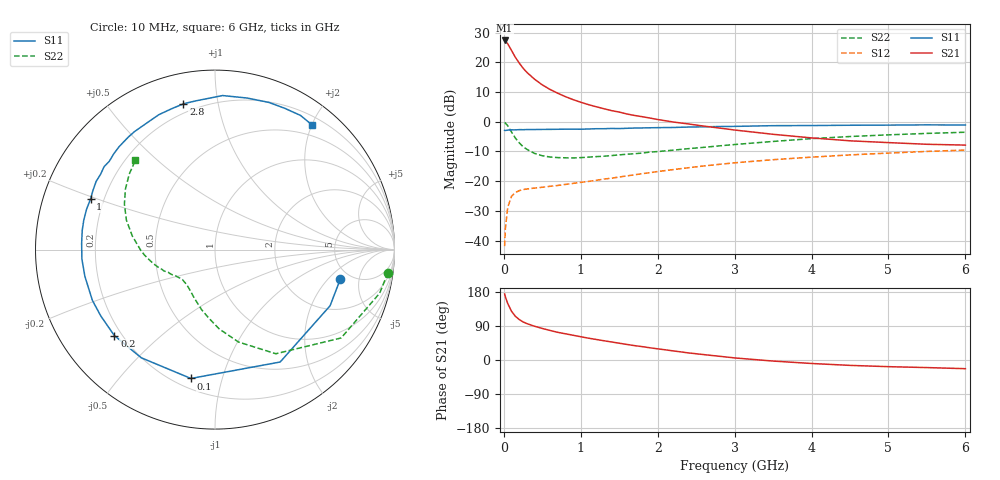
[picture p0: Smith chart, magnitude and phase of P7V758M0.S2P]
! SIEMENS Small Signal Semiconductors
! BFP196
! Si NPN RF Bipolar Junction Transistor in SOT143
! VCE = 0.75 V  IC = 8 mA
! Common Emitter S-Parameters:  May  1996
# GHz  S  MA  R  50
!  f  S11  S21  S12  S22
! GHz  MAG  ANG  MAG  ANG  MAG  ANG  MAG  ANG
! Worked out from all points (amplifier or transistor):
!   36 points, 10 MHz to 6 GHz, reference 50 ohm
!   highest |S21| = 27.3 dB at 10 MHz (marker M1)
!   |S21| within 3 dB of that: start of sweep to 91.81 MHz
!   unconditionally stable (mu >= 1): 904.2 MHz to end of sweep
!   at 250 MHz: K = 0.36, MSG = 20.4 dB, |S12| = -22.8 dB
!   at 1.4 GHz: K = 1.16, MAG = 8.9 dB, |S12| = -19.0 dB
!   at 6 GHz: K = 1.04, MAG = -0.3 dB, |S12| = -9.5 dB
!   S11 on the Smith chart (normalised r, x): 10 MHz: 4.08, -2.79; 100 MHz: 0.26, -0.80; 200 MHz: 0.17, -0.36; 1 GHz: 0.15, +0.19; 2.8 GHz: 0.15, +0.80; 6 GHz: 0.32, +2.00
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0.01  0.717 -13.4  23.25 174.3  0.0081 83.3  0.9719 -7.6
0.02  0.7135 -26.0  22.61 166.7  0.016 78.2  0.9492 -14.8
0.05  0.7239 -59.9  20.45 149.4  0.0363 62.4  0.8582 -35.0
0.1  0.7304 -100.6  15.77 128.5  0.056 45.1  0.6721 -59.7
0.15  0.7295 -124.3  12.1 115.3  0.0646 35.7  0.5315 -75.7
0.2  0.7375 -139.5  9.699 106.8  0.0694 30.7  0.4423 -87.0
0.25  0.7359 -149.9  7.95 100.5  0.0724 27.8  0.3808 -95.6
0.3  0.7394 -157.5  6.754 96.0  0.0741 26.5  0.3433 -102.5
0.4  0.7401 -168.4  5.175 89.0  0.0768 25.3  0.2935 -113.2
0.5  0.7434 -175.9  4.163 83.3  0.0792 25.8  0.268 -120.7
0.6  0.7439 177.3  3.494 78.0  0.0822 26.8  0.2555 -126.2
0.7  0.7475 171.7  3.017 73.1  0.0849 27.9  0.2497 -130.8
0.8  0.7494 167.3  2.643 69.2  0.0884 29.2  0.2476 -134.6
1  0.7486 157.9  2.126 61.4  0.0957 32.0  0.2495 -139.9
1.1  0.7557 154.1  1.94 57.6  0.0993 32.7  0.2542 -142.1
1.6  0.7765 136.6  1.35 41.0  0.1229 36.3  0.2845 -152.1
2.2  0.8009 118.5  0.991 24.1  0.1569 35.8  0.3329 -163.1
2.8  0.8312 102.2  0.784 9.9  0.1922 31.8  0.3931 -175.4
3.5  0.8593 87.2  0.615 -2.8  0.2303 24.7  0.4666 170.7
4.5  0.8732 69.9  0.478 -14.2  0.277 13.9  0.5644 153.4
5.5  0.8864 57.5  0.418 -20.0  0.317 2.9  0.6367 138.6
6  0.8805 52.1  0.405 -22.9  0.3342 -3.2  0.6662 131.8
